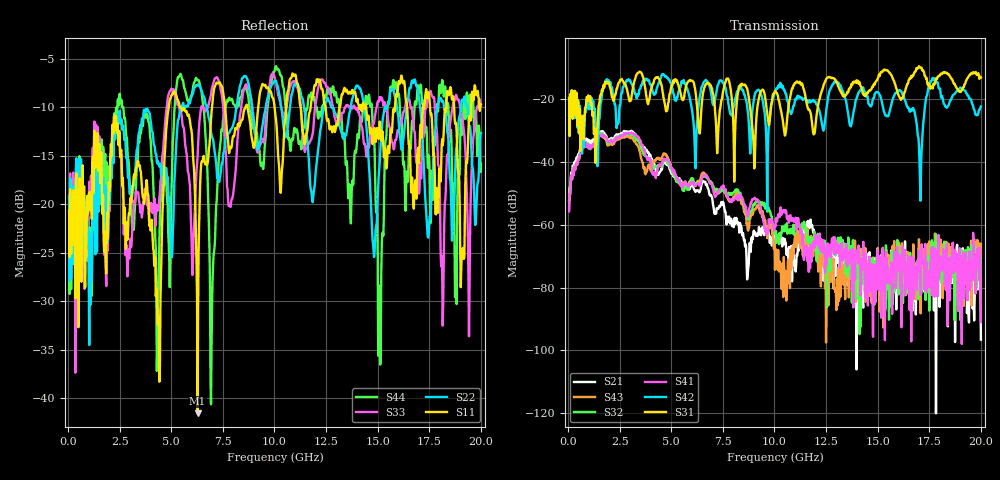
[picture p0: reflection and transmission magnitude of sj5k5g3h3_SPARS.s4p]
! FILE: E:\users\goganessyan\GBX_Backplane\FR408_backplane\1m_INBOUND_FEXT\sj5k5g3h3_SPARS.s4p
# MHZ S RI R 50.00
! FREQ  S11  S12  S13  S14
!  S21  S22  S23  S24
!  S31  S32  S33  S34
!  S41  S42  S43  S44
!  REAL  IMAG  REAL  IMAG  REAL  IMAG  REAL  IMAG
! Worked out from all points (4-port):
!   799 points, 50 MHz to 20 GHz, reference 50 ohm
!   strongest paths, dB at 50 MHz, 5.025 GHz, 10.03 GHz, 15.03 GHz, 20 GHz:
!     S31: -19.7, -15.6, -17.5, -13.2, -13.2
!     S42: -19.7, -16.1, -17.7, -17.9, -22.4
!     S41: -55.8, -42.4, -60.4, -75.3, -91.1
!     S32: -52.2, -42.6, -62.6, -79.8, -70.6
!     S43: -54.7, -42.2, -74.3, -74.2, -70.4
!     S21: -52.3, -43.8, -63.4, -75.6, -96.6
!   lowest |S11| = -41.5 dB at 6.275 GHz (marker M1), VSWR 1.02, Z = 50.6 - j0.628 ohm
!   |S11| at or under -10 dB: start of sweep to 4.875 GHz; 5.456 GHz to 6.976 GHz (1.52 GHz wide, 24.4 % of centre); 14.44 GHz to 15.84 GHz (1.395 GHz wide, 9.22 % of centre)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
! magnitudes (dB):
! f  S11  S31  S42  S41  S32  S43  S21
! 50 MHz  -20.7  -19.7  -19.7  -55.8  -52.2  -54.7  -52.3
! 6.275 GHz  -41.5  -24.5  -25.2  -47.0  -46.5  -46.3  -49.1
! 6.95 GHz  -10.5  -16.4  -19.1  -46.9  -46.9  -46.9  -50.9
! 10.38 GHz  -16.1  -25.8  -15.7  -55.9  -60.5  -72.4  -66.9
! 15.1 GHz  -11.5  -12.7  -18.6  -71.0  -74.8  -87.7  -78.4
! 15.7 GHz  -12.4  -12.9  -20.6  -88.4  -80.8  -69.3  -76.7
! 20 GHz  -9.7  -13.2  -22.4  -91.1  -70.6  -70.4  -96.6
